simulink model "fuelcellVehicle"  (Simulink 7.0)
settings: Solver=ode45  StartTime=0.0  StopTime=10.0  RelTol=1e-3
InitFcn:
  | t_Start=tic;
StopFcn:
  | t_elapsed=toc(t_Start);
  | fuel_cons=(1000*(fueltank_simple1_std(end,1)/fueltank_simple1_std(end,3)))/(chassis_simple4_std(end,2)/100000);
  | 
  | disp(' ')
  | disp(['Time Elapsed: ' num2str(round(100*t_elapsed)/100) 's'])
  | disp(['Fuel Consumption: ' num2str(round(1000*fuel_cons)/1000) 'L/100km'])
undefined symbols (not defined in the file or in its folder): computed_mass, DC, fuelcellVehicle, Left, levelinit, slcm
libraries: simulink x11
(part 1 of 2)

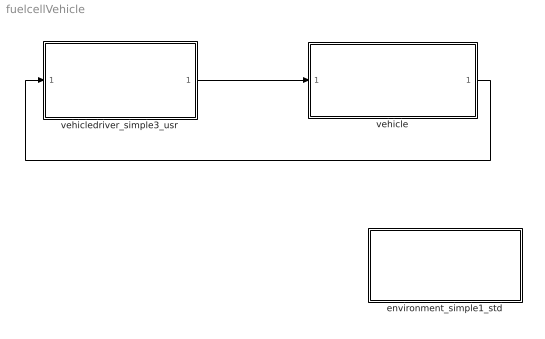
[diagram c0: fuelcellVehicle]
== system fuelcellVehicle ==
  environment_simple1_std : Subsystem  mask{Tamb=300, Pamb=101300}
      mask prompts: Tamb "Ambient Temperature [K]"; Pamb "Ambient Pressure [Pa]"
      mask help: Environment settings
  vehicle : Subsystem
  vehicledriver_simple3_usr : Subsystem  mask{Kp_driver=0.3, Ki_driver=0.02}
      mask prompts: Kp_driver "Proportional Gain"; Ki_driver "Integral Gain"
      mask help: Driver model
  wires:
  vehicledriver_simple3_usr/1(driver cmd out) -> vehicle/1(In1)
  vehicle/1(Out1) -> vehicledriver_simple3_usr/1(vehicle fb in)

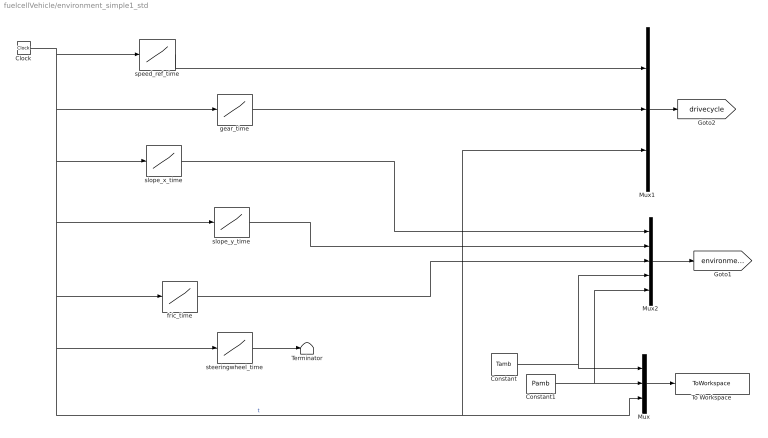
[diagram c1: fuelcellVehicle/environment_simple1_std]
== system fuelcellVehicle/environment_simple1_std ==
  Clock : Clock
  Constant : Constant  Value=Tamb  OutDataType=sfix(16)  OutScaling=2^0
  Constant1 : Constant  Value=Pamb  OutDataType=sfix(16)  OutScaling=2^0
  Mux : Mux  Inputs=3
  Mux1 : Mux  Inputs=3
  Mux2 : Mux  Inputs=5
  Terminator : Terminator
  To Workspace : ToWorkspace  VariableName=environment_simple1_std  SampleTime=-1  SaveFormat=Array
  fric_time : Lookup  InputValues=DC.time  Table=DC.fric  OutDataType=sfix(16)  OutScaling=2^0
  gear_time : Lookup  InputValues=DC.time  Table=DC.gearnr  OutDataType=sfix(16)  OutScaling=2^0
  slope_x_time : Lookup  InputValues=DC.time  Table=DC.slope_x  OutDataType=sfix(16)  OutScaling=2^0
  slope_y_time : Lookup  InputValues=DC.time  Table=DC.slope_y  OutDataType=sfix(16)  OutScaling=2^0
  speed_ref_time : Lookup  InputValues=DC.time  Table=DC.speed  OutDataType=sfix(16)  OutScaling=2^0
  steeringwheel_time : Lookup  InputValues=DC.time  Table=DC.steeringwheel  OutDataType=sfix(16)  OutScaling=2^0
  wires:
  Constant1/1 -> Mux/2, Mux2/5
  Constant/1 -> Mux/1, Mux2/4
  Mux/1 -> To Workspace/1
  Clock/1 -> speed_ref_time/1, gear_time/1, slope_x_time/1, slope_y_time/1, fric_time/1, Mux/3, Mux1/3, steeringwheel_time/1  "t"
  Mux1/1 -> [drivecycle]
  speed_ref_time/1 -> Mux1/1
  gear_time/1 -> Mux1/2
  slope_x_time/1 -> Mux2/1
  slope_y_time/1 -> Mux2/2
  fric_time/1 -> Mux2/3
  steeringwheel_time/1 -> Terminator/1
  Mux2/1 -> [environment]

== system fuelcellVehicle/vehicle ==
  In1 : Inport  OutDataType=sfix(16)  OutScaling=2^0
  Bus Creator : BusCreator  Orientation=up  Inputs=1
  Bus Creator1 : BusCreator  Orientation=up
  Bus Selector : BusSelector  Orientation=down  OutputSignals=fuelcell,electricmotor,chassis
  Ground : Ground
  Terminator : Terminator
  buffer_simple1_std : Subsystem
  chassis_simple4_std : Subsystem  InitFcn=computed_mass=calc_total_mass;
  controller_fuelcell1_usr : Subsystem  mask{SOCref=0.5}
      mask prompts: SOCref "SOC reference (0-1)"
      mask help: Main Controller
  electricmotor_quasistatic2_std : Subsystem
  electricsplit_simple1_std : Subsystem
  fuelcell_simple1_usr : Subsystem
  fueltank_simple1_std : Subsystem  mask{tanksize=??, level=100, fueldensity=??, Hf=??}
      mask prompts: tanksize "Size of fuel tank  [l]"; level "Level in tank [%]"; fueldensity "Fuel density [kg/m3]"; Hf "Specific Calorific Value [MJ/kg]"
      mask help: This is an ideal internal combustion engine component
  Out1 : Outport  OutDataType=sfix(16)  OutScaling=2^0
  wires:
  In1/1 -> controller_fuelcell1_usr/1(driver cmd in)
  controller_fuelcell1_usr/1(vehicle fb out) -> Out1/1
  electricmotor_quasistatic2_std/2(mech out [Nm]) -> chassis_simple4_std/2(mech in [Nm])
  chassis_simple4_std/2(mech fb out [rad/s]) -> electricmotor_quasistatic2_std/3(mech fb in [rad/s])
  fueltank_simple1_std/1(chem SCV out [MJ/kg]) -> fuelcell_simple1_usr/2(chem SCV in [MJ/kg])
  fuelcell_simple1_usr/3(chem fb out [kg/s]) -> fueltank_simple1_std/1(chem fb in [kg/s])
  controller_fuelcell1_usr/2(cmd out) -> Bus Selector/1
  Bus Creator1/1 -> controller_fuelcell1_usr/2(sensor in)
  Bus Creator/1 -> chassis_simple4_std/3(el in [V])
  chassis_simple4_std/3(el fb out [A]) -> Terminator/1
  Ground/1 -> Bus Creator/1  "voltage [V]"
  Bus Selector/1 -> fuelcell_simple1_usr/1(cmd)  "<fuelcell>"
  Bus Selector/2 -> electricmotor_quasistatic2_std/1(cmd in)  "<electricmotor>"
  Bus Selector/3 -> chassis_simple4_std/1(cmd)  "<chassis>"
  fuelcell_simple1_usr/1(sensor out) -> Bus Creator1/1
  electricmotor_quasistatic2_std/1(sensor out) -> Bus Creator1/2
  chassis_simple4_std/1(sensor out) -> Bus Creator1/3
  buffer_simple1_std/2(el out [V]) -> electricsplit_simple1_std/3(el split in [V])
  electricsplit_simple1_std/1(el out [V]) -> electricmotor_quasistatic2_std/2(el in [V])
  electricsplit_simple1_std/3(el split out [A]) -> buffer_simple1_std/1(el fb in [A])
  buffer_simple1_std/1(sensor out) -> Bus Creator1/4
  fuelcell_simple1_usr/2(el out [V]) -> electricsplit_simple1_std/1(el in [A])
  electricmotor_quasistatic2_std/3(el fb out [A]) -> electricsplit_simple1_std/2(el fb in [A])
  electricsplit_simple1_std/2(el fb out [V]) -> fuelcell_simple1_usr/3(el fb in [V])

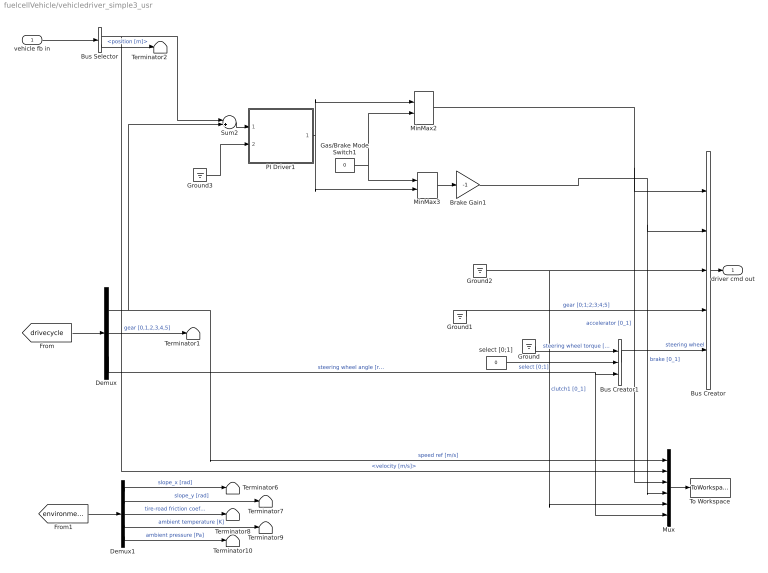
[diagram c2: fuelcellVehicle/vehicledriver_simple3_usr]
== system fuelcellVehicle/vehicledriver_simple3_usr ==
  vehicle fb in : Inport  OutDataType=sfix(16)  OutScaling=2^0
  Brake Gain1 : Gain  Gain=-1  ParameterDataType=sfix(16)  ParameterScaling=2^0  OutDataType=sfix(16)  OutScaling=2^0
  Bus Creator : BusCreator  Inputs=5
  Bus Creator1 : BusCreator  Inputs=3
  Bus Selector : BusSelector  OutputSignals=chassis.velocity [m/s],chassis.position [m]
  Demux : Demux  Outputs=3
  Demux1 : Demux  Outputs=5
  Gas/Brake Mode Switch1 : Constant  Value=0  OutDataType=sfix(16)  OutScaling=2^0
  Ground{,1..3} (4 alike) : Ground
  MinMax2 : MinMax  Function=max  Inputs=2  OutDataType=sfix(16)  OutScaling=2^0
  MinMax3 : MinMax  Inputs=2  OutDataType=sfix(16)  OutScaling=2^0
  Mux : Mux  Inputs=6
  PI Driver1 : Subsystem
  Sum2 : Sum  Inputs=-+  OutDataType=sfix(16)  OutScaling=2^0
  Terminator{1..2,6..10} (7 alike) : Terminator
  To Workspace : ToWorkspace  VariableName=driver_simple1_std  SampleTime=-1  SaveFormat=Array
  select [0;1] : Constant  Value=0  OutDataType=sfix(16)  OutScaling=2^0
  driver cmd out : Outport  OutDataType=sfix(16)  OutScaling=2^0
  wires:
  Ground3/1 -> PI Driver1/2(PI reset)
  select [0;1]/1 -> Bus Creator1/2  "select [0;1]"
  Demux/1 -> Sum2/2, Mux/1  "speed ref [m/s]"
  Demux/3 -> Bus Creator1/3, Mux/6  "steering wheel angle [rad]"
  [drivecycle] -> Demux/1
  Demux/2 -> Terminator1/1  "gear [0,1,2,3,4,5]"
  Demux1/5 -> Terminator10/1  "ambient pressure [Pa]"
  Demux1/4 -> Terminator9/1  "ambient temperature [K]"
  Demux1/1 -> Terminator6/1  "slope_x [rad]"
  Demux1/3 -> Terminator8/1  "tire-road friction coefficient [-]"
  [environment] -> Demux1/1
  Demux1/2 -> Terminator7/1  "slope_y [rad]"
  Bus Creator/1 -> driver cmd out/1
  Ground/1 -> Bus Creator1/1  "steering wheel torque [Nm]"
  Mux/1 -> To Workspace/1
  Bus Creator1/1 -> Bus Creator/5  "steering wheel"
  Ground1/1 -> Bus Creator/4  "gear [0;1;2;3;4;5]"
  Ground2/1 -> Bus Creator/3, Mux/5  "clutch1 [0_1]"
  MinMax2/1 -> Bus Creator/1, Mux/3  "accelerator [0_1]"
  Gas/Brake Mode Switch1/1 -> MinMax3/1, MinMax2/2
  MinMax3/1 -> Brake Gain1/1
  PI Driver1/1(PI out) -> MinMax3/2, MinMax2/1
  Brake Gain1/1 -> Bus Creator/2, Mux/4  "brake [0_1]"
  Sum2/1 -> PI Driver1/1(PI input)
  vehicle fb in/1 -> Bus Selector/1
  Bus Selector/1 -> Mux/2, Sum2/1  "<velocity [m/s]>"
  Bus Selector/2 -> Terminator2/1  "<position [m]>"

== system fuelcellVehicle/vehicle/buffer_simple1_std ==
  el fb in [A] : Inport  OutDataType=sfix(16)  OutScaling=2^0
  Model Info1 : Subsystem  LoadFcn=slcm LoadBlock;  InitFcn=slcm('UpdateAllCMBlocksInThisModelInit')  mask(CMBlock){InitialSaveTempField=, InitialBlockCM=None, BlockCM=None, Frame=on, SaveTempField=, DisplayStringWithTags=This model level is fixed. Place parameters in the subsystem masks, not on the top level., MaskDisplayString=This model level is fixed. Place parameters in the\nsubsystem masks, not on the top level., HorizontalTextAlignment=Left, LeftAlignmentValue=0.02, SourceBlockDiagram=fuelcellVehicle, TagMaxNumber=20, CMTag1=, CMTag2=, CMTag3=, CMTag4=, CMTag5=, CMTag6=, CMTag7=, CMTag8=, CMTag9=, CMTag10=, CMTag11=, CMTag12=, CMTag13=, CMTag14=, CMTag15=, CMTag16=, CMTag17=, CMTag18=, CMTag19=, CMTag20=}
      mask help: This block allows revision control information to be displayed within the model.
  buffer : Subsystem  mask{mass=??, Emax=??, Ri=??, Kvol=??, SOCinit=0.5}
      mask prompts: mass "Mass [kg]"; Emax "Maximum Energy level [J]"; Ri "Inner Resistance [Ohm]"; Kvol "Maximum voltage [V]"; SOCinit "SOC inital value"
      mask help: Electric buffer model
  local controller : Subsystem  mask{Kvol_c=??, Ri_c=??, Emax_c=??, SOCinit_c=??}
      mask prompts: Kvol_c "Maximum voltage [V]"; Ri_c "Inner Resistance [Ohm]"; Emax_c "Battery Energy Maxlevel [J]"; SOCinit_c "SOC initial level"
      mask help: Local controller for electric buffer
  sensor out : Outport  OutDataType=sfix(16)  OutScaling=2^0
  el out [V] : Outport  Port=2  OutDataType=sfix(16)  OutScaling=2^0
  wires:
  buffer/2(el out [V]) -> el out [V]/1
  local controller/1(sensor out) -> sensor out/1
  el fb in [A]/1 -> buffer/2(el fb in [A])
  buffer/1(sensor out) -> local controller/1(sensor in)
  local controller/2(ctrl) -> buffer/1(ctrl)

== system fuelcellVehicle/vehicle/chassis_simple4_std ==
  cmd : Inport  OutDataType=sfix(16)  OutScaling=2^0
  mech in [Nm] : Inport  Port=2  OutDataType=sfix(16)  OutScaling=2^0
  el in [V] : Inport  Port=3  OutDataType=sfix(16)  OutScaling=2^0
  chassis : Subsystem  mask{mass=??, nop=1, passengerweight=80, cargo=0, w_init=1, tirespec='205/55R16' %Modify this if needed, e=??, Cd=??, Af=??, rho=1.2, finalgear=3}
      mask prompts: mass "Chassis Mass [kg]"; nop "Number of passengers"; passengerweight "Weight of avg. passenger (kg)"; cargo "Cargo load (kg)"; w_init "Initial velocity [rad/s]"; tirespec "Tire specification (ex: '205/55R16')"; e "Rolling resistance coeff rear"; Cd "Air resistance cd (-)"; Af "Air resistance frontal area (m2)"; rho "Air density (kg/m3)"; finalgear "Final gear"
      mask help: Chassis model template
      mask init:
      | r=tireradius(tirespec);
  local controller : Subsystem
  sensor out : Outport  OutDataType=sfix(16)  OutScaling=2^0
  mech fb out [rad/s] : Outport  Port=2  OutDataType=sfix(16)  OutScaling=2^0
  el fb out [A] : Outport  Port=3  OutDataType=sfix(16)  OutScaling=2^0
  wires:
  local controller/2(ctrl) -> chassis/1(ctrl)
  chassis/2(mech fb out [rad/s]) -> mech fb out [rad/s]/1
  mech in [Nm]/1 -> chassis/2(mech in [Nm])
  chassis/1(sensor out) -> local controller/2(sensor in)
  local controller/1(sensor out) -> sensor out/1
  cmd/1 -> local controller/1(cmd in)
  el in [V]/1 -> chassis/3(el in [V])
  chassis/3(el fb out [A]) -> el fb out [A]/1

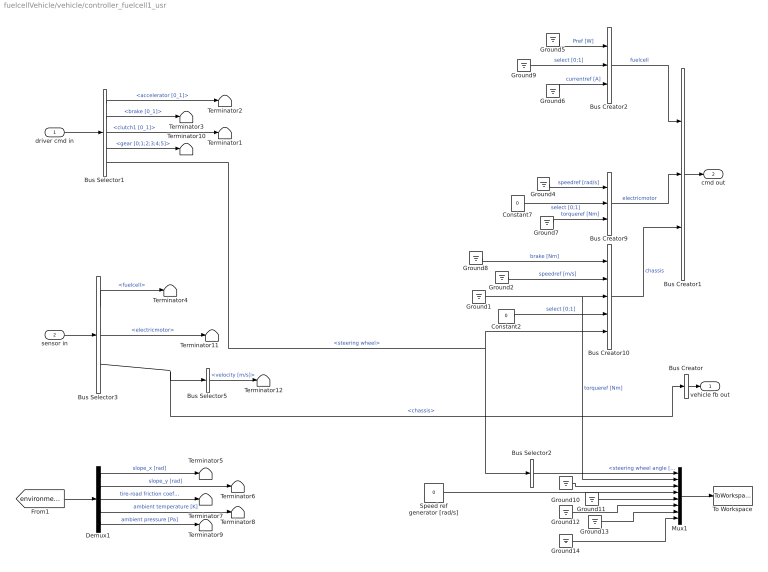
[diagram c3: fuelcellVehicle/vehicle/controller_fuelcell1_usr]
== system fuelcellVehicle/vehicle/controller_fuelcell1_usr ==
  driver cmd in : Inport  OutDataType=sfix(16)  OutScaling=2^0
  sensor in : Inport  Port=2  OutDataType=sfix(16)  OutScaling=2^0
  Bus Creator : BusCreator  Inputs=1
  Bus Creator1 : BusCreator  Inputs=3
  Bus Creator10 : BusCreator  Inputs=5
  Bus Creator2 : BusCreator  Inputs=3
  Bus Creator9 : BusCreator  Inputs=3
  Bus Selector1 : BusSelector  OutputSignals=accelerator [0_1],brake [0_1],clutch1 [0_1],gear [0;1;2;3;4;5],steering wheel
  Bus Selector2 : BusSelector  OutputSignals=steering wheel angle [rad]
  Bus Selector3 : BusSelector  OutputSignals=fuelcell,electricmotor,chassis
  Bus Selector5 : BusSelector  OutputSignals=velocity [m/s]
  Constant2 : Constant  Value=0  OutDataType=sfix(16)  OutScaling=2^0
  Constant7 : Constant  Value=0  OutDataType=sfix(16)  OutScaling=2^0
  Demux1 : Demux  Outputs=5
  Ground{1..2,4..14} (13 alike) : Ground
  Mux1 : Mux  Inputs=8
  Speed ref generator [rad/s] : Constant  Value=0  OutDataType=sfix(16)  OutScaling=2^0
  Terminator{1..12} (12 alike) : Terminator
  To Workspace : ToWorkspace  VariableName=controller_fuelcell1_usr  SampleTime=-1  SaveFormat=Array
  vehicle fb out : Outport  OutDataType=sfix(16)  OutScaling=2^0
  cmd out : Outport  Port=2  OutDataType=sfix(16)  OutScaling=2^0
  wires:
  Demux1/5 -> Terminator9/1  "ambient pressure [Pa]"
  Demux1/4 -> Terminator8/1  "ambient temperature [K]"
  Demux1/1 -> Terminator5/1  "slope_x [rad]"
  Demux1/3 -> Terminator7/1  "tire-road friction coefficient [-]"
  [environment] -> Demux1/1
  Demux1/2 -> Terminator6/1  "slope_y [rad]"
  Speed ref generator [rad/s]/1 -> Mux1/4
  Bus Selector2/1 -> Mux1/1  "<steering wheel angle [rad]>"
  Mux1/1 -> To Workspace/1
  Constant2/1 -> Bus Creator10/4  "select [0;1]"
  Ground1/1 -> Mux1/2, Bus Creator10/3  "torqueref [Nm]"
  Ground2/1 -> Bus Creator10/2  "speedref [m/s]"
  Bus Creator10/1 -> Bus Creator1/3  "chassis"
  Bus Creator9/1 -> Bus Creator1/2  "electricmotor"
  Constant7/1 -> Bus Creator9/2  "select [0;1]"
  Ground4/1 -> Bus Creator9/1  "speedref [rad/s]"
  Bus Selector3/3 -> Bus Creator/1, Bus Selector5/1  "<chassis>"
  Bus Selector3/1 -> Terminator4/1  "<fuelcell>"
  Bus Selector3/2 -> Terminator11/1  "<electricmotor>"
  sensor in/1 -> Bus Selector3/1
  driver cmd in/1 -> Bus Selector1/1
  Bus Selector1/5 -> Bus Selector2/1, Bus Creator10/5  "<steering wheel>"
  Bus Creator/1 -> vehicle fb out/1
  Bus Creator1/1 -> cmd out/1
  Bus Creator2/1 -> Bus Creator1/1  "fuelcell"
  Ground5/1 -> Bus Creator2/1  "Pref [W]"
  Ground6/1 -> Bus Creator2/3  "currentref [A]"
  Bus Selector1/2 -> Terminator3/1  "<brake [0_1]>"
  Bus Selector1/1 -> Terminator2/1  "<accelerator [0_1]>"
  Bus Selector1/3 -> Terminator1/1  "<clutch1 [0_1]>"
  Bus Selector1/4 -> Terminator10/1  "<gear [0;1;2;3;4;5]>"
  Ground7/1 -> Bus Creator9/3  "torqueref [Nm]"
  Ground8/1 -> Bus Creator10/1  "brake [Nm]"
  Ground9/1 -> Bus Creator2/2  "select [0;1]"
  Bus Selector5/1 -> Terminator12/1  "<velocity [m/s]>"
  Ground10/1 -> Mux1/3
  Ground11/1 -> Mux1/5
  Ground12/1 -> Mux1/6
  Ground13/1 -> Mux1/7
  Ground14/1 -> Mux1/8

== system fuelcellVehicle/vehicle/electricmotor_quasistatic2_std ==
  cmd in : Inport  OutDataType=sfix(16)  OutScaling=2^0
  el in [V] : Inport  Port=2  OutDataType=sfix(16)  OutScaling=2^0
  mech fb in [rad/s] : Inport  Port=3  OutDataType=sfix(16)  OutScaling=2^0
  electricmotor : Subsystem  mask{mass=??, inertia=??, ka=??, ki=??, R=??}
      mask prompts: mass "Mass (kg)"; inertia "Inertia (kg*m^2)"; ka "Motor torque constant (Nm/A) (slightly smaller than voltage/speed constant)"; ki "Voltage/speed constant"; R "Resistance (ohm)"
  local controller : Subsystem  mask{kac=??, kic=??, Rc=??, Pmax=??, Kp=10, Ki=1}
      mask prompts: kac "Motor torque constant (Nm/A) (slightly smaller than voltage/speed constant)"; kic "Voltage/speed constant"; Rc "Motor resistance (ohm)"; Pmax "Max power (kW)"; Kp "Speed controller (Kp)"; Ki "Speed controller (Ki)"
  sensor out : Outport  OutDataType=sfix(16)  OutScaling=2^0
  mech out [Nm] : Outport  Port=2  OutDataType=sfix(16)  OutScaling=2^0
  el fb out [A] : Outport  Port=3  OutDataType=sfix(16)  OutScaling=2^0
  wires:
  local controller/1(sensor out) -> sensor out/1
  electricmotor/2(mech power out [Nm]) -> mech out [Nm]/1
  electricmotor/3(el fb out [A]) -> el fb out [A]/1
  cmd in/1 -> local controller/1(cmd in)
  mech fb in [rad/s]/1 -> electricmotor/3(mech fb in [rad/s])
  el in [V]/1 -> electricmotor/2(el power in [V])
  electricmotor/1(sensor out) -> local controller/2(sensor in)
  local controller/2(ctrl out) -> electricmotor/1(ctrl in)

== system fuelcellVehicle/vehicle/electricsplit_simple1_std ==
  el in [A] : Inport  OutDataType=sfix(16)  OutScaling=2^0
  el fb in [A] : Inport  Port=2  OutDataType=sfix(16)  OutScaling=2^0
  el split in [V] : Inport  Port=3  OutDataType=sfix(16)  OutScaling=2^0
  Model Info1 : simulink/Model-Wide Utilities/Model Info  SystemSampleTime=-1  InitialBlockCM=None  BlockCM=None  Frame=on  DisplayStringWithTags=This model level is fixed. Place parameters in the subsystem masks, not on the top level.  HorizontalTextAlignment=Left  LeftAlignmentValue=0.02  SourceBlockDiagram=fuelcellVehicle  TagMaxNumber=20
  electricsplit : Subsystem  mask{mass=0}
      mask prompts: mass "Mass [kg]"
      mask help: Electric buffer template model
  local controller : Subsystem
  el out [V] : Outport  OutDataType=sfix(16)  OutScaling=2^0
  el fb out [V] : Outport  Port=2  OutDataType=sfix(16)  OutScaling=2^0
  el split out [A] : Outport  Port=3  OutDataType=sfix(16)  OutScaling=2^0
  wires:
  local controller/1(ctrl) -> electricsplit/1(ctrl)
  electricsplit/1(sensor out) -> local controller/1(sensor in)
  el split in [V]/1 -> electricsplit/4(el split in [V])
  electricsplit/4(el split out [A]) -> el split out [A]/1
  el in [A]/1 -> electricsplit/2(el in [A])
  el fb in [A]/1 -> electricsplit/3(el fb in [A])
  electricsplit/3(el fb out [V]) -> el fb out [V]/1
  electricsplit/2(el out [V]) -> el out [V]/1

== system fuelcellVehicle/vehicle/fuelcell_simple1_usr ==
  cmd : Inport  OutDataType=sfix(16)  OutScaling=2^0
  chem SCV in [MJ/kg] : Inport  Port=2  OutDataType=sfix(16)  OutScaling=2^0
  el fb in [V] : Inport  Port=3  OutDataType=sfix(16)  OutScaling=2^0
  Model Info1 : Subsystem  LoadFcn=slcm LoadBlock;  InitFcn=slcm('UpdateAllCMBlocksInThisModelInit')  mask(CMBlock){InitialSaveTempField=, InitialBlockCM=None, BlockCM=None, Frame=on, SaveTempField=, DisplayStringWithTags=This model level is fixed. Place parameters in the subsystem masks, not on the top level., MaskDisplayString=This model level is fixed. Place parameters in the\nsubsystem masks, not on the top level., HorizontalTextAlignment=Left, LeftAlignmentValue=0.02, SourceBlockDiagram=fuelcellVehicle, TagMaxNumber=20, CMTag1=, CMTag2=, CMTag3=, CMTag4=, CMTag5=, CMTag6=, CMTag7=, CMTag8=, CMTag9=, CMTag10=, CMTag11=, CMTag12=, CMTag13=, CMTag14=, CMTag15=, CMTag16=, CMTag17=, CMTag18=, CMTag19=, CMTag20=}
      mask help: This block allows revision control information to be displayed within the model.
  fuelcell : Subsystem  mask{mass=??}
      mask prompts: mass "Mass [kg]"
      mask help: Internal combustion engine template model
  local controller : Subsystem
  sensor out : Outport  OutDataType=sfix(16)  OutScaling=2^0
  el out [V] : Outport  Port=2  OutDataType=sfix(16)  OutScaling=2^0
  chem fb out [kg/s] : Outport  Port=3  OutDataType=sfix(16)  OutScaling=2^0
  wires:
  fuelcell/2(el power out [A]) -> el out [V]/1
  el fb in [V]/1 -> fuelcell/3(el fb in [V])
  fuelcell/1(sensor out) -> local controller/2(sensor in)
  local controller/1(sensor out) -> sensor out/1
  cmd/1 -> local controller/1(cmd)
  local controller/2(ctrl) -> fuelcell/1(ctrl)
  fuelcell/3(chem fb out [kg/s]) -> chem fb out [kg/s]/1
  chem SCV in [MJ/kg]/1 -> fuelcell/2(chem SCV in [MJ/kg])

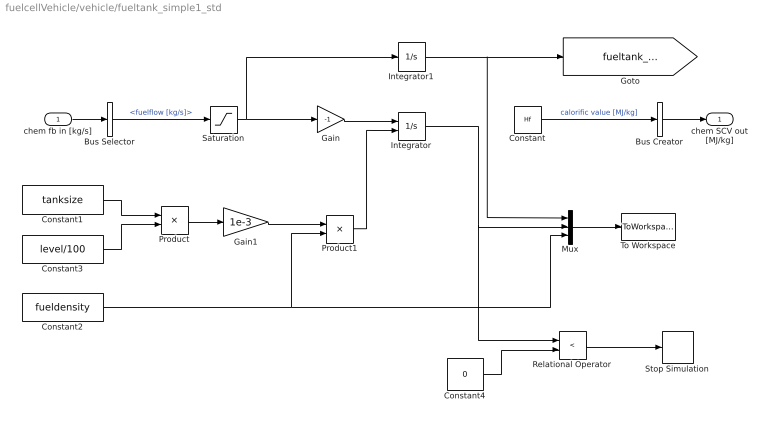
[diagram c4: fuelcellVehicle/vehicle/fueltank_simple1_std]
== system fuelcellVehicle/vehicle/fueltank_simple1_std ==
  chem fb in [kg/s] : Inport  OutDataType=sfix(16)  OutScaling=2^0
  Bus Creator : BusCreator  Inputs=1
  Bus Selector : BusSelector  OutputSignals=fuelflow [kg/s]
  Constant : Constant  Value=Hf  OutDataType=sfix(16)  OutScaling=2^0
  Constant1 : Constant  Value=tanksize  OutDataType=sfix(16)  OutScaling=2^0
  Constant2 : Constant  Value=fueldensity  OutDataType=sfix(16)  OutScaling=2^0
  Constant3 : Constant  Value=level/100  OutDataType=sfix(16)  OutScaling=2^0
  Constant4 : Constant  Value=0  OutDataType=sfix(16)  OutScaling=2^0
  Gain : Gain  Gain=-1  ParameterDataType=sfix(16)  ParameterScaling=2^0  OutDataType=sfix(16)  OutScaling=2^0
  Gain1 : Gain  Gain=1e-3  ParameterDataType=sfix(16)  ParameterScaling=2^0  OutDataType=sfix(16)  OutScaling=2^0
  Integrator : Integrator  InitialConditionSource=external  InitialCondition=levelinit
  Integrator1 : Integrator
  Mux : Mux  Inputs=3
  Product : Product  OutDataType=sfix(16)  OutScaling=2^0
  Product1 : Product  OutDataType=sfix(16)  OutScaling=2^0
  Relational Operator : RelationalOperator  Operator=<  LogicOutDataTypeMode=boolean
  Saturation : Saturate  UpperLimit=inf  LowerLimit=0
  Stop Simulation : Stop
  To Workspace : ToWorkspace  VariableName=fueltank_simple1_std  SampleTime=-1  SaveFormat=Array
  chem SCV out [MJ/kg] : Outport  OutDataType=sfix(16)  OutScaling=2^0
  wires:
  chem fb in [kg/s]/1 -> Bus Selector/1
  Constant/1 -> Bus Creator/1  "calorific value [MJ/kg]"
  Gain/1 -> Integrator/1
  Bus Selector/1 -> Saturation/1  "<fuelflow [kg/s]>"
  Mux/1 -> To Workspace/1
  Integrator1/1 -> Mux/1, [fueltank_weight_reduction]
  Integrator/1 -> Mux/2, Relational Operator/1
  Bus Creator/1 -> chem SCV out [MJ/kg]/1
  Constant1/1 -> Product/1
  Constant3/1 -> Product/2
  Constant2/1 -> Mux/3, Product1/2
  Product/1 -> Gain1/1
  Product1/1 -> Integrator/2
  Gain1/1 -> Product1/1
  Constant4/1 -> Relational Operator/2
  Relational Operator/1 -> Stop Simulation/1
  Saturation/1 -> Gain/1, Integrator1/1

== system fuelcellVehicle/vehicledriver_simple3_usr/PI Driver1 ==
  PI input : Inport  OutDataType=sfix(16)  OutScaling=2^0
  PI reset : Inport  Port=2  OutDataType=sfix(16)  OutScaling=2^0
  Integrator : Integrator  ExternalReset=either  LimitOutput=on  UpperSaturationLimit=30  LowerSaturationLimit=0
  Ki : Gain  Gain=Ki_driver  ParameterDataType=sfix(16)  ParameterScaling=2^0  OutDataType=sfix(16)  OutScaling=2^0
  Kp : Gain  Gain=Kp_driver  ParameterDataType=sfix(16)  ParameterScaling=2^0  OutDataType=sfix(16)  OutScaling=2^0
  Saturation : Saturate  UpperLimit=1  LowerLimit=-1
  Sum : Sum  Inputs=|++  OutDataType=sfix(16)  OutScaling=2^0
  PI out : Outport  OutDataType=sfix(16)  OutScaling=2^0
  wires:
  Kp/1 -> Sum/1
  PI reset/1 -> Integrator/2
  Saturation/1 -> PI out/1
  Sum/1 -> Saturation/1
  Ki/1 -> Sum/2
  Integrator/1 -> Ki/1
  PI input/1 -> Kp/1, Integrator/1

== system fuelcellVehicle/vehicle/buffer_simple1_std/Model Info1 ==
  EmptySubsystem : Subsystem

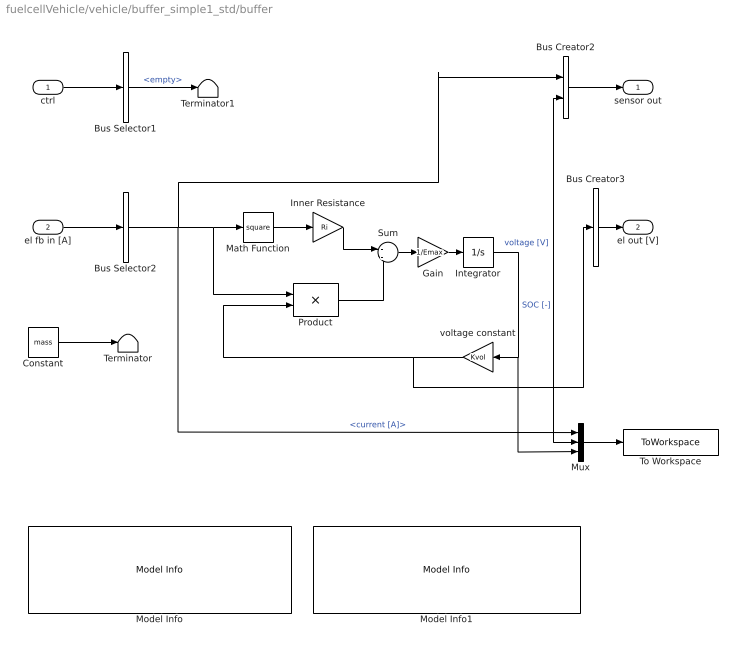
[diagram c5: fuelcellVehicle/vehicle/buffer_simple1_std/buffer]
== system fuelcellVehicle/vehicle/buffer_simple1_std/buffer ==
  ctrl : Inport  OutDataType=sfix(16)  OutScaling=2^0
  el fb in [A] : Inport  Port=2  OutDataType=sfix(16)  OutScaling=2^0
  Bus Creator2 : BusCreator  Inputs=2
  Bus Creator3 : BusCreator  Inputs=1
  Bus Selector1 : BusSelector  OutputSignals=empty
  Bus Selector2 : BusSelector  OutputSignals=current [A]
  Constant : Constant  Value=mass  OutDataType=sfix(16)  OutScaling=2^0
  Gain : Gain  Gain=1/Emax  ParameterDataType=sfix(16)  ParameterScaling=2^0  OutDataType=sfix(16)  OutScaling=2^0
  Inner Resistance : Gain  Gain=Ri  ParameterDataType=sfix(16)  ParameterScaling=2^0  OutDataType=sfix(16)  OutScaling=2^0
  Integrator : Integrator  InitialCondition=SOCinit  LimitOutput=on  UpperSaturationLimit=1  LowerSaturationLimit=0
  Math Function : Math  Operator=square  OutDataType=sfix(16)  OutScaling=2^0
  Model Info : simulink/Model-Wide Utilities/Model Info  SystemSampleTime=-1  InitialBlockCM=None  BlockCM=None  Frame=on  DisplayStringWithTags=|  HorizontalTextAlignment=Left  LeftAlignmentValue=0.02  SourceBlockDiagram=fuelcellVehicle  TagMaxNumber=20
      | Modified: %<ModifiedDate>
      | 
      | The nodes "ctrl" and "sensor out" must conform 
      | with the corresponding nodes of the local controller. 
      | The other nodes are fixed.
  Model Info1 : simulink/Model-Wide Utilities/Model Info  SystemSampleTime=-1  InitialBlockCM=None  BlockCM=None  Frame=on  DisplayStringWithTags=Your own comments!  HorizontalTextAlignment=Left  LeftAlignmentValue=0.02  SourceBlockDiagram=fuelcellVehicle  TagMaxNumber=20
  Mux : Mux  Inputs=3
  Product : Product  OutDataType=sfix(16)  OutScaling=2^0
  Sum : Sum  Inputs=-|-  OutDataType=sfix(16)  OutScaling=2^0
  Terminator : Terminator
  Terminator1 : Terminator
  To Workspace : ToWorkspace  VariableName=buffer_simple1_std  SampleTime=-1  SaveFormat=Array
  voltage constant : Gain  Orientation=left  Gain=Kvol  ParameterDataType=sfix(16)  ParameterScaling=2^0  OutDataType=sfix(16)  OutScaling=2^0
  sensor out : Outport  OutDataType=sfix(16)  OutScaling=2^0
  el out [V] : Outport  Port=2  OutDataType=sfix(16)  OutScaling=2^0
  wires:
  Bus Selector1/1 -> Terminator1/1  "<empty>"
  ctrl/1 -> Bus Selector1/1
  Bus Creator2/1 -> sensor out/1
  Bus Creator3/1 -> el out [V]/1
  Bus Selector2/1 -> Bus Creator2/1, Math Function/1, Product/1, Mux/1  "<current [A]>"
  el fb in [A]/1 -> Bus Selector2/1
  Constant/1 -> Terminator/1
  Integrator/1 -> voltage constant/1, Mux/3  "SOC [-]"
  Gain/1 -> Integrator/1
  Math Function/1 -> Inner Resistance/1
  voltage constant/1 -> Product/2, Bus Creator3/1, Bus Creator2/2, Mux/2  "voltage [V]"
  Inner Resistance/1 -> Sum/1
  Product/1 -> Sum/2
  Sum/1 -> Gain/1
  Mux/1 -> To Workspace/1

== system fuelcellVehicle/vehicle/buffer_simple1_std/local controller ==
  sensor in : Inport  OutDataType=sfix(16)  OutScaling=2^0
  Bus Creator1 : BusCreator  Inputs=1
  Bus Creator2 : BusCreator  Inputs=3
  Bus Selector2 : BusSelector  OutputSignals=current [A],voltage [V]
  Ground : Ground
  Model Info : simulink/Model-Wide Utilities/Model Info  SystemSampleTime=-1  InitialBlockCM=None  BlockCM=None  Frame=on  DisplayStringWithTags=|  HorizontalTextAlignment=Left  LeftAlignmentValue=0.02  SourceBlockDiagram=fuelcellVehicle  TagMaxNumber=20
      | Modified: %<ModifiedDate>
      | 
      | The nodes "cmd in" and "sensor out" are fixed.
      | The nodes "sensor in" and "ctrl", however, 
      | may be adjusted arbitrarily since the local controller is 
      | made specifically for a certain component model.
  Model Info1 : simulink/Model-Wide Utilities/Model Info  SystemSampleTime=-1  InitialBlockCM=None  BlockCM=None  Frame=on  DisplayStringWithTags=Your own comments!  HorizontalTextAlignment=Left  LeftAlignmentValue=0.02  SourceBlockDiagram=fuelcellVehicle  TagMaxNumber=20
  SOC estimator : Subsystem
  sensor out : Outport  OutDataType=sfix(16)  OutScaling=2^0
  ctrl : Outport  Port=2  OutDataType=sfix(16)  OutScaling=2^0
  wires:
  Bus Selector2/2 -> Bus Creator2/3  "<voltage [V]>"
  Ground/1 -> Bus Creator1/1  "empty"
  Bus Creator1/1 -> ctrl/1
  Bus Creator2/1 -> sensor out/1  "buffer"
  Bus Selector2/1 -> Bus Creator2/1, SOC estimator/1(current in)  "<current [A]>"
  sensor in/1 -> Bus Selector2/1
  SOC estimator/1(SOC) -> Bus Creator2/2  "SOC [-]"

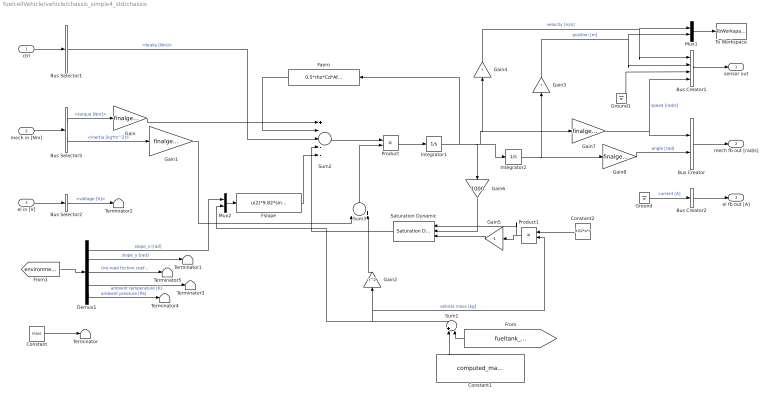
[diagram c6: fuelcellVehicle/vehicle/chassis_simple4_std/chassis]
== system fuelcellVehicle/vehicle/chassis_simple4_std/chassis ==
  ctrl : Inport  OutDataType=sfix(16)  OutScaling=2^0
  mech in [Nm] : Inport  Port=2  OutDataType=sfix(16)  OutScaling=2^0
  el in [V] : Inport  Port=3  OutDataType=sfix(16)  OutScaling=2^0
  Bus Creator : BusCreator  Inputs=2
  Bus Creator1 : BusCreator
  Bus Creator2 : BusCreator  Inputs=1
  Bus Selector1 : BusSelector  OutputSignals=brake [Nm]
  Bus Selector2 : BusSelector  OutputSignals=voltage [V]
  Bus Selector5 : BusSelector  OutputSignals=torque [Nm],inertia [kg*m^2]
  Constant : Constant  Value=mass  OutDataType=sfix(16)  OutScaling=2^0
  Constant1 : Constant  Orientation=up  Value=computed_mass  OutDataType=sfix(16)  OutScaling=2^0
  Constant2 : Constant  Orientation=left  Value=9.82*e*r  OutDataType=sfix(16)  OutScaling=2^0
  Demux1 : Demux  Outputs=5
  Faero : Fcn  Orientation=left  Expr=0.5*rho*Cd*Af*u^2*r^3
  Fslope : Fcn  Expr=u(2)*9.82*sin(u(1))
  Gain : Gain  Gain=finalgear  ParameterDataType=sfix(16)  ParameterScaling=2^0  OutDataType=sfix(16)  OutScaling=2^0
  Gain1 : Gain  Gain=finalgear^2  ParameterDataType=sfix(16)  ParameterScaling=2^0  OutDataType=sfix(16)  OutScaling=2^0
  Gain2 : Gain  Orientation=up  Gain=r^2  ParameterDataType=sfix(16)  ParameterScaling=2^0  OutDataType=sfix(16)  OutScaling=2^0
  Gain3 : Gain  Orientation=up  Gain=r  ParameterDataType=sfix(16)  ParameterScaling=2^0  OutDataType=sfix(16)  OutScaling=2^0
  Gain4 : Gain  Orientation=up  Gain=r  ParameterDataType=sfix(16)  ParameterScaling=2^0  OutDataType=sfix(16)  OutScaling=2^0
  Gain5 : Gain  Orientation=left  Gain=-1  ParameterDataType=sfix(16)  ParameterScaling=2^0  OutDataType=sfix(16)  OutScaling=2^0
  Gain6 : Gain  Orientation=down  Gain=1000  ParameterDataType=sfix(16)  ParameterScaling=2^0  OutDataType=sfix(16)  OutScaling=2^0
  Gain7 : Gain  Gain=finalgear  ParameterDataType=sfix(16)  ParameterScaling=2^0  OutDataType=sfix(16)  OutScaling=2^0
  Gain8 : Gain  Gain=finalgear  ParameterDataType=sfix(16)  ParameterScaling=2^0  OutDataType=sfix(16)  OutScaling=2^0
  Ground : Ground
  Ground1 : Ground
  Integrator1 : Integrator  InitialCondition=w_init
  Integrator2 : Integrator
  Mux1 : Mux  Inputs=2
  Mux2 : Mux  Inputs=2
  Product : Product  Inputs=*/  OutDataType=sfix(16)  OutScaling=2^0
  Product1 : Product  Orientation=left  Inputs=**  OutDataType=sfix(16)  OutScaling=2^0
  Saturation Dynamic : simulink/Discontinuities/Saturation Dynamic  Orientation=left  SystemSampleTime=-1  OutMin=[]  OutMax=[]  OutDataTypeStr=Inherit: Same as second input  OutDataType=sfix(16)  OutScaling=2^-10  DoSatur=off
  Sum1 : Sum  Orientation=up  Inputs=+|-  OutDataType=sfix(16)  OutScaling=2^0
  Sum2 : Sum  Inputs=+----  OutDataType=sfix(16)  OutScaling=2^0
  Sum3 : Sum  Orientation=up  OutDataType=sfix(16)  OutScaling=2^0
  Terminator{,1..5} (6 alike) : Terminator
  To Workspace : ToWorkspace  VariableName=chassis_simple4_std  SampleTime=-1  SaveFormat=Array
  sensor out : Outport  OutDataType=sfix(16)  OutScaling=2^0
  mech fb out [rad/s] : Outport  Port=2  OutDataType=sfix(16)  OutScaling=2^0
  el fb out [A] : Outport  Port=3  OutDataType=sfix(16)  OutScaling=2^0
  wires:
  Ground1/1 -> Bus Creator1/3
  Mux2/1 -> Fslope/1
  Bus Selector5/2 -> Gain1/1  "<inertia [kg*m^2]>"
  Bus Selector5/1 -> Gain/1  "<torque [Nm]>"
  Bus Creator/1 -> mech fb out [rad/s]/1
  mech in [Nm]/1 -> Bus Selector5/1
  Constant/1 -> Terminator/1
  Bus Creator1/1 -> sensor out/1
  Mux1/1 -> To Workspace/1
  ctrl/1 -> Bus Selector1/1
  Bus Selector2/1 -> Terminator2/1  "<voltage [V]>"
  el in [V]/1 -> Bus Selector2/1
  Bus Creator2/1 -> el fb out [A]/1
  Ground/1 -> Bus Creator2/1  "current [A]"
  Constant1/1 -> Sum1/1
  Sum1/1 -> Mux2/2, Gain2/1, Product1/2  "vehicle mass [kg]"
  [fueltank_weight_reduction] -> Sum1/2
  Demux1/2 -> Terminator1/1  "slope_y [rad]"
  [environment] -> Demux1/1
  Demux1/4 -> Terminator3/1  "ambient temperature [K]"
  Demux1/5 -> Terminator4/1  "ambient pressure [Pa]"
  Demux1/3 -> Terminator5/1  "tire-road friction coefficient [-]"
  Bus Selector1/1 -> Sum2/3  "<brake [Nm]>"
  Demux1/1 -> Mux2/1  "slope_x [rad]"
  Gain/1 -> Sum2/1
  Integrator1/1 -> Faero/1, Integrator2/1, Gain4/1, Gain7/1, Gain6/1
  Faero/1 -> Sum2/2
  Fslope/1 -> Sum2/5
  Integrator2/1 -> Gain3/1, Gain8/1
  Gain2/1 -> Sum3/2
  Gain1/1 -> Sum3/1
  Sum3/1 -> Product/2
  Product/1 -> Integrator1/1
  Sum2/1 -> Product/1
  Gain3/1 -> Mux1/2, Bus Creator1/2  "position [m]"
  Gain4/1 -> Mux1/1, Bus Creator1/1  "velocity [m/s]"
  Saturation Dynamic/1 -> Sum2/4
  Product1/1 -> Gain5/1, Saturation Dynamic/1
  Constant2/1 -> Product1/1
  Gain5/1 -> Saturation Dynamic/3
  Gain6/1 -> Saturation Dynamic/2
  Gain7/1 -> Bus Creator/1, Bus Creator1/4  "speed [rad/s]"
  Gain8/1 -> Bus Creator/2  "angle [rad]"

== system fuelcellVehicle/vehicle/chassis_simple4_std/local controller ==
  cmd in : Inport  OutDataType=sfix(16)  OutScaling=2^0
  sensor in : Inport  Port=2  OutDataType=sfix(16)  OutScaling=2^0
  Bus Creator1 : BusCreator  Inputs=1
  Bus Creator2 : BusCreator  Inputs=2
  Bus Selector1 : BusSelector  OutputSignals=velocity [m/s],position [m]
  Bus Selector2 : BusSelector  OutputSignals=brake [Nm]
  sensor out : Outport  OutDataType=sfix(16)  OutScaling=2^0
  ctrl : Outport  Port=2  OutDataType=sfix(16)  OutScaling=2^0
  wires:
  Bus Selector2/1 -> Bus Creator1/1  "<brake [Nm]>"
  Bus Creator1/1 -> ctrl/1
  Bus Creator2/1 -> sensor out/1  "chassis"
  sensor in/1 -> Bus Selector1/1
  Bus Selector1/1 -> Bus Creator2/1  "<velocity [m/s]>"
  cmd in/1 -> Bus Selector2/1
  Bus Selector1/2 -> Bus Creator2/2  "<position [m]>"

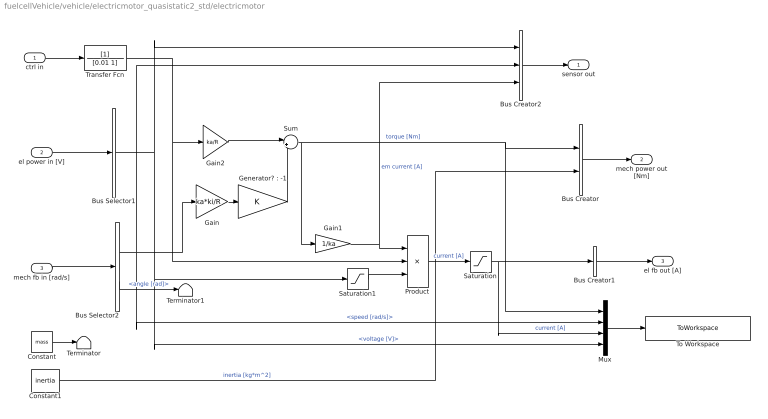
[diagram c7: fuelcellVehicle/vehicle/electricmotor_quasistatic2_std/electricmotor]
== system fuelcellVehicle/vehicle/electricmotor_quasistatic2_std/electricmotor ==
  ctrl in : Inport  OutDataType=sfix(16)  OutScaling=2^0
  el power in [V] : Inport  Port=2  OutDataType=sfix(16)  OutScaling=2^0
  mech fb in [rad/s] : Inport  Port=3  OutDataType=sfix(16)  OutScaling=2^0
  Bus Creator : BusCreator  Inputs=2
  Bus Creator1 : BusCreator  Inputs=1
  Bus Creator2 : BusCreator  Inputs=3
  Bus Selector1 : BusSelector  OutputSignals=voltage [V]
  Bus Selector2 : BusSelector  OutputSignals=speed [rad/s],angle [rad]
  Constant : Constant  Value=mass  OutDataType=sfix(16)  OutScaling=2^0
  Constant1 : Constant  Value=inertia  OutDataType=sfix(16)  OutScaling=2^0
  Gain : Gain  Gain=ka*ki/R  ParameterDataType=sfix(16)  ParameterScaling=2^0  OutDataType=sfix(16)  OutScaling=2^0
  Gain1 : Gain  Gain=1/ka  ParameterDataType=sfix(16)  ParameterScaling=2^0  OutDataType=sfix(16)  OutScaling=2^0
  Gain2 : Gain  Gain=ka/R  ParameterDataType=sfix(16)  ParameterScaling=2^0  OutDataType=sfix(16)  OutScaling=2^0
  "Generator? : -1" : Gain  ParameterDataType=sfix(16)  ParameterScaling=2^0  OutDataType=sfix(16)  OutScaling=2^0
  Mux : Mux
  Product : Product  Inputs=**/  OutDataType=sfix(16)  OutScaling=2^0
  Saturation : Saturate  UpperLimit=300  LowerLimit=-300
  Saturation1 : Saturate  UpperLimit=inf  LowerLimit=0.1
  Sum : Sum  Inputs=|+-  OutDataType=sfix(16)  OutScaling=2^0
  Terminator : Terminator
  Terminator1 : Terminator
  To Workspace : ToWorkspace  VariableName=electricmotor_quasistatic2_std  SampleTime=-1  SaveFormat=Array
  Transfer Fcn : TransferFcn  Denominator=[0.01 1]
  sensor out : Outport  OutDataType=sfix(16)  OutScaling=2^0
  mech power out [Nm] : Outport  Port=2  OutDataType=sfix(16)  OutScaling=2^0
  el fb out [A] : Outport  Port=3  OutDataType=sfix(16)  OutScaling=2^0
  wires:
  Bus Creator1/1 -> el fb out [A]/1
  Bus Selector2/2 -> Terminator1/1  "<angle [rad]>"
  Bus Creator/1 -> mech power out [Nm]/1
  el power in [V]/1 -> Bus Selector1/1
  Constant/1 -> Terminator/1
  mech fb in [rad/s]/1 -> Bus Selector2/1
  ctrl in/1 -> Transfer Fcn/1
  Bus Selector2/1 -> Mux/2, Gain/1, Bus Creator2/2  "<speed [rad/s]>"
  Bus Selector1/1 -> Bus Creator2/1, Mux/4, Saturation1/1  "<voltage [V]>"
  Product/1 -> Saturation/1  "current [A]"
  Mux/1 -> To Workspace/1
  Bus Creator2/1 -> sensor out/1
  Constant1/1 -> Bus Creator/2  "inertia [kg*m^2]"
  Gain/1 -> "Generator? : -1"/1
  Gain1/1 -> Bus Creator2/3, Product/1  "em current [A]"
  Transfer Fcn/1 -> Gain2/1, Product/2
  Gain2/1 -> Sum/1
  Sum/1 -> Gain1/1, Mux/1, Bus Creator/1  "torque [Nm]"
  "Generator? : -1"/1 -> Sum/2
  Saturation/1 -> Bus Creator1/1, Mux/3  "current [A]"
  Saturation1/1 -> Product/3

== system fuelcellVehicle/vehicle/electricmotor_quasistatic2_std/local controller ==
  cmd in : Inport  OutDataType=sfix(16)  OutScaling=2^0
  sensor in : Inport  Port=2  OutDataType=sfix(16)  OutScaling=2^0
  Bus Creator1 : BusCreator  Inputs=1
  Bus Creator2 : BusCreator  Inputs=3
  Bus Selector1 : BusSelector  OutputSignals=speedref [rad/s],select [0;1],torqueref [Nm]
  Bus Selector3 : BusSelector  OutputSignals=voltage [V],speed [rad/s],em current [A]
  Gain : Gain  ParameterDataType=sfix(16)  ParameterScaling=2^0  OutDataType=sfix(16)  OutScaling=2^0
  Selector : Subsystem
  Speedcontroller : Subsystem
  Torquecontroller : Subsystem
  sensor out : Outport  OutDataType=sfix(16)  OutScaling=2^0
  ctrl out : Outport  Port=2  OutDataType=sfix(16)  OutScaling=2^0
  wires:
  cmd in/1 -> Bus Selector1/1
  Bus Selector1/1 -> Speedcontroller/1(Speedref)  "<speedref [rad/s]>"
  Bus Selector1/2 -> Selector/3(Select)  "<select [0;1]>"
  Bus Creator2/1 -> sensor out/1  "electricmotor"
  Selector/1(Ctrl) -> Bus Creator2/1, Bus Creator1/1  "voltage [V]"
  sensor in/1 -> Bus Selector3/1
  Bus Selector3/1 -> Selector/4(BatVolt)  "<voltage [V]>"
  Bus Selector3/3 -> Gain/1  "<em current [A]>"
  Bus Creator1/1 -> ctrl out/1
  Bus Selector1/3 -> Torquecontroller/1(Torqueref)  "<torqueref [Nm]>"
  Bus Selector3/2 -> Speedcontroller/2(Speed), Bus Creator2/2, Torquecontroller/2(Speed), Selector/5(Speed [rad/s])  "<speed [rad/s]>"
  Torquecontroller/1(Volt) -> Selector/2(TorqueCtrl)
  Speedcontroller/1(Volt) -> Selector/1(SpeedCtrl)
  Gain/1 -> Bus Creator2/3  "current [A]"

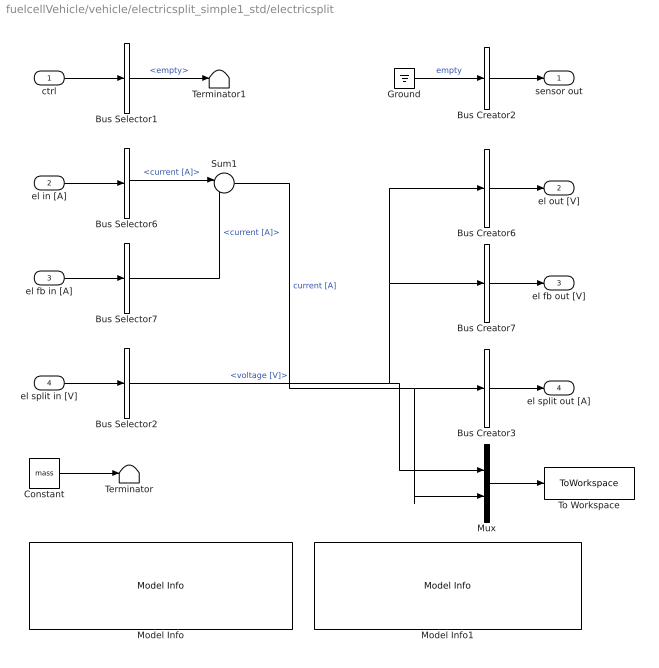
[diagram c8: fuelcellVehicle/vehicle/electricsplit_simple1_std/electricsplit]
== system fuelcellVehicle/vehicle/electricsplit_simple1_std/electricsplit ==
  ctrl : Inport  OutDataType=sfix(16)  OutScaling=2^0
  el in [A] : Inport  Port=2  OutDataType=sfix(16)  OutScaling=2^0
  el fb in [A] : Inport  Port=3  OutDataType=sfix(16)  OutScaling=2^0
  el split in [V] : Inport  Port=4  OutDataType=sfix(16)  OutScaling=2^0
  Bus Creator{2..3,6..7} (4 alike) : BusCreator  Inputs=1
  Bus Selector1 : BusSelector  OutputSignals=empty
  Bus Selector2 : BusSelector  OutputSignals=voltage [V]
  Bus Selector6 : BusSelector  OutputSignals=current [A]
  Bus Selector7 : BusSelector  OutputSignals=current [A]
  Constant : Constant  Value=mass  OutDataType=sfix(16)  OutScaling=2^0
  Ground : Ground
  Model Info : simulink/Model-Wide Utilities/Model Info  SystemSampleTime=-1  InitialBlockCM=None  BlockCM=None  Frame=on  DisplayStringWithTags=|  HorizontalTextAlignment=Left  LeftAlignmentValue=0.02  SourceBlockDiagram=fuelcellVehicle  TagMaxNumber=20
      | Modified: %<ModifiedDate>
      | 
      | The nodes "ctrl" and "sensor out" must conform 
      | with the corresponding nodes of the local controller. 
      | The other nodes are fixed.
  Model Info1 : simulink/Model-Wide Utilities/Model Info  SystemSampleTime=-1  InitialBlockCM=None  BlockCM=None  Frame=on  DisplayStringWithTags=Your own comments!  HorizontalTextAlignment=Left  LeftAlignmentValue=0.02  SourceBlockDiagram=fuelcellVehicle  TagMaxNumber=20
  Mux : Mux  Inputs=2
  Sum1 : Sum  Inputs=|-+  OutDataType=sfix(16)  OutScaling=2^0
  Terminator : Terminator
  Terminator1 : Terminator
  To Workspace : ToWorkspace  VariableName=electricsplit_simple1_std  SampleTime=-1  SaveFormat=Array
  sensor out : Outport  OutDataType=sfix(16)  OutScaling=2^0
  el out [V] : Outport  Port=2  OutDataType=sfix(16)  OutScaling=2^0
  el fb out [V] : Outport  Port=3  OutDataType=sfix(16)  OutScaling=2^0
  el split out [A] : Outport  Port=4  OutDataType=sfix(16)  OutScaling=2^0
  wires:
  Constant/1 -> Terminator/1
  Bus Selector2/1 -> Bus Creator6/1, Bus Creator7/1, Mux/1  "<voltage [V]>"
  Bus Creator3/1 -> el split out [A]/1
  Bus Creator2/1 -> sensor out/1
  ctrl/1 -> Bus Selector1/1
  Bus Selector1/1 -> Terminator1/1  "<empty>"
  el in [A]/1 -> Bus Selector6/1
  Bus Selector6/1 -> Sum1/1  "<current [A]>"
  Bus Creator6/1 -> el out [V]/1
  el fb in [A]/1 -> Bus Selector7/1
  Bus Selector7/1 -> Sum1/2  "<current [A]>"
  Bus Creator7/1 -> el fb out [V]/1
  Sum1/1 -> Bus Creator3/1, Mux/2  "current [A]"
  el split in [V]/1 -> Bus Selector2/1
  Ground/1 -> Bus Creator2/1  "empty"
  Mux/1 -> To Workspace/1

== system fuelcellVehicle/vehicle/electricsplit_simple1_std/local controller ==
  sensor in : Inport  OutDataType=sfix(16)  OutScaling=2^0
  Bus Creator1 : BusCreator  Inputs=1
  Bus Selector2 : BusSelector  OutputSignals=empty
  Ground : Ground
  Model Info : simulink/Model-Wide Utilities/Model Info  SystemSampleTime=-1  InitialBlockCM=None  BlockCM=None  Frame=on  DisplayStringWithTags=|  HorizontalTextAlignment=Left  LeftAlignmentValue=0.02  SourceBlockDiagram=fuelcellVehicle  TagMaxNumber=20
      | Modified: %<ModifiedDate>
      | The node "sensor out" is fixed.
      | The nodes "sensor in" and "ctrl", however, 
      | may be adjusted arbitrarily since the local controller is 
      | made specifically for a certain component model.
  Model Info1 : simulink/Model-Wide Utilities/Model Info  SystemSampleTime=-1  InitialBlockCM=None  BlockCM=None  Frame=on  DisplayStringWithTags=Your own comments!  HorizontalTextAlignment=Left  LeftAlignmentValue=0.02  SourceBlockDiagram=fuelcellVehicle  TagMaxNumber=20
  Terminator1 : Terminator
  ctrl : Outport  OutDataType=sfix(16)  OutScaling=2^0
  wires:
  Bus Creator1/1 -> ctrl/1
  Ground/1 -> Bus Creator1/1  "empty"
  sensor in/1 -> Bus Selector2/1
  Bus Selector2/1 -> Terminator1/1  "<empty>"

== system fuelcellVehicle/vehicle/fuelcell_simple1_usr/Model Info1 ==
  EmptySubsystem : Subsystem

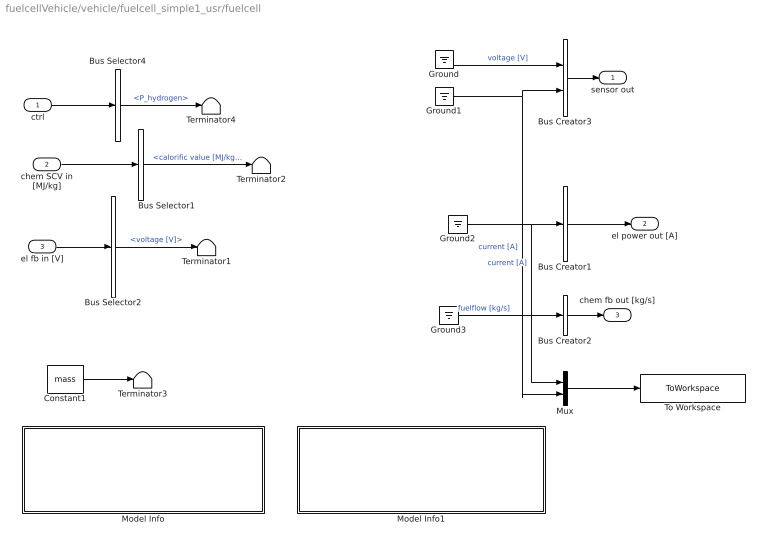
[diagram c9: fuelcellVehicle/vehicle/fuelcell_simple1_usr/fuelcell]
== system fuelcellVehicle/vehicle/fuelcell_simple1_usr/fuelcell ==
  ctrl : Inport  OutDataType=sfix(16)  OutScaling=2^0
  chem SCV in [MJ/kg] : Inport  Port=2  OutDataType=sfix(16)  OutScaling=2^0
  el fb in [V] : Inport  Port=3  OutDataType=sfix(16)  OutScaling=2^0
  Bus Creator1 : BusCreator  Inputs=1
  Bus Creator2 : BusCreator  Inputs=1
  Bus Creator3 : BusCreator  Inputs=2
  Bus Selector1 : BusSelector  OutputSignals=calorific value [MJ/kg]
  Bus Selector2 : BusSelector  OutputSignals=voltage [V]
  Bus Selector4 : BusSelector  OutputSignals=P_hydrogen
  Constant1 : Constant  Value=mass  OutDataType=sfix(16)  OutScaling=2^0
  Ground{,1..3} (4 alike) : Ground
  Model Info : Subsystem  LoadFcn=slcm LoadBlock;  InitFcn=slcm('UpdateAllCMBlocksInThisModelInit')  mask(CMBlock){InitialSaveTempField=, InitialBlockCM=None, BlockCM=None, Frame=on, SaveTempField=, DisplayStringWithTags=Modified: %<ModifiedDate>  The nodes "ctrl" and "sensor out" must conform  with the corresponding nodes of the local controller.  The other nodes are fixed., MaskDisplayString=Modified: Fri Dec  3 15:47:20 2010\n\nThe nodes "ctrl" and "sensor out" must conform \nwith the corresponding nodes of the local controller. \nThe other nodes are fixed., HorizontalTextAlignment=Left, LeftAlignmentValue=0.02, SourceBlockDiagram=fuelcellVehicle, TagMaxNumber=20, CMTag1=, CMTag2=, CMTag3=, CMTag4=, CMTag5=, CMTag6=, CMTag7=, CMTag8=, CMTag9=, CMTag10=, CMTag11=, CMTag12=, CMTag13=, CMTag14=, CMTag15=, CMTag16=, CMTag17=, CMTag18=, CMTag19=, CMTag20=}
      mask help: This block allows revision control information to be displayed within the model.
  Model Info1 : Subsystem  LoadFcn=slcm LoadBlock;  InitFcn=slcm('UpdateAllCMBlocksInThisModelInit')  mask(CMBlock){InitialSaveTempField=, InitialBlockCM=None, BlockCM=None, Frame=on, SaveTempField=, DisplayStringWithTags=Your own comments!, MaskDisplayString=Your own comments!, HorizontalTextAlignment=Left, LeftAlignmentValue=0.02, SourceBlockDiagram=fuelcellVehicle, TagMaxNumber=20, CMTag1=, CMTag2=, CMTag3=, CMTag4=, CMTag5=, CMTag6=, CMTag7=, CMTag8=, CMTag9=, CMTag10=, CMTag11=, CMTag12=, CMTag13=, CMTag14=, CMTag15=, CMTag16=, CMTag17=, CMTag18=, CMTag19=, CMTag20=}
      mask help: This block allows revision control information to be displayed within the model.
  Mux : Mux  Inputs=2
  Terminator{1..4} (4 alike) : Terminator
  To Workspace : ToWorkspace  VariableName=fuelcell_simple1_usr  SampleTime=-1  SaveFormat=Array
  sensor out : Outport  OutDataType=sfix(16)  OutScaling=2^0
  el power out [A] : Outport  Port=2  OutDataType=sfix(16)  OutScaling=2^0
  chem fb out [kg/s] : Outport  Port=3  OutDataType=sfix(16)  OutScaling=2^0
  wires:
  el fb in [V]/1 -> Bus Selector2/1
  Bus Creator1/1 -> el power out [A]/1
  Bus Creator3/1 -> sensor out/1
  ctrl/1 -> Bus Selector4/1
  chem SCV in [MJ/kg]/1 -> Bus Selector1/1
  Ground3/1 -> Bus Creator2/1  "fuelflow [kg/s]"
  Constant1/1 -> Terminator3/1
  Bus Creator2/1 -> chem fb out [kg/s]/1
  Mux/1 -> To Workspace/1
  Bus Selector4/1 -> Terminator4/1  "<P_hydrogen>"
  Bus Selector2/1 -> Terminator1/1  "<voltage [V]>"
  Bus Selector1/1 -> Terminator2/1  "<calorific value [MJ/kg]>"
  Ground/1 -> Bus Creator3/1  "voltage [V]"
  Ground1/1 -> Bus Creator3/2, Mux/2  "current [A]"
  Ground2/1 -> Bus Creator1/1, Mux/1  "current [A]"

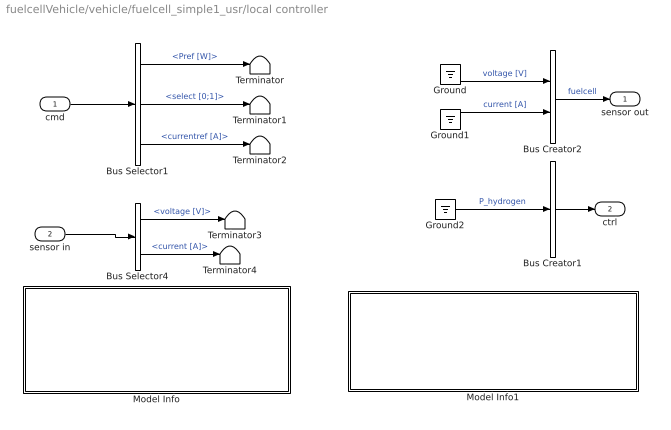
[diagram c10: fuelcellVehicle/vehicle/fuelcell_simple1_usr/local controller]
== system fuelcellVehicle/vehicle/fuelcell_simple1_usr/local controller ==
  cmd : Inport  OutDataType=sfix(16)  OutScaling=2^0
  sensor in : Inport  Port=2  OutDataType=sfix(16)  OutScaling=2^0
  Bus Creator1 : BusCreator  Inputs=1
  Bus Creator2 : BusCreator  Inputs=2
  Bus Selector1 : BusSelector  OutputSignals=Pref [W],select [0;1],currentref [A]
  Bus Selector4 : BusSelector  OutputSignals=voltage [V],current [A]
  Ground : Ground
  Ground1 : Ground
  Ground2 : Ground
  Model Info : Subsystem  LoadFcn=slcm LoadBlock;  InitFcn=slcm('UpdateAllCMBlocksInThisModelInit')  mask(CMBlock){InitialSaveTempField=, InitialBlockCM=None, BlockCM=None, Frame=on, SaveTempField=, DisplayStringWithTags=Modified: %<ModifiedDate> The nodes "cmd" and "sensor out" are fixed. The "select" signal defines whether the upper  (=1) or lower (=0) signal is used. The nodes "sensor in" and "ctrl", however,  may be adjusted arbitrarily since the local  controller is made specifically for a certain  component model., MaskDisplayString=Modified: Fri Dec  3 15:47:20 2010\nThe nodes "cmd" and "sensor out" are fixed.\nThe "select" signal defines whether the upper \n(=1) or lower (=0) signal is used.\nThe nodes "sensor in" and "ctrl", however, \nmay be adjusted arbitrarily since the local \ncontroller is made specifically for a certain \ncomponent model., HorizontalTextAlignment=Left, LeftAlignmentValue=0.02, SourceBlockDiagram=fuelcellVehicle, TagMaxNumber=20, CMTag1=, CMTag2=, CMTag3=, CMTag4=, CMTag5=, CMTag6=, CMTag7=, CMTag8=, CMTag9=, CMTag10=, CMTag11=, CMTag12=, CMTag13=, CMTag14=, CMTag15=, CMTag16=, CMTag17=, CMTag18=, CMTag19=, CMTag20=}
      mask help: This block allows revision control information to be displayed within the model.
  Model Info1 : Subsystem  LoadFcn=slcm LoadBlock;  InitFcn=slcm('UpdateAllCMBlocksInThisModelInit')  mask(CMBlock){InitialSaveTempField=, InitialBlockCM=None, BlockCM=None, Frame=on, SaveTempField=, DisplayStringWithTags=Your own comments!, MaskDisplayString=Your own comments!, HorizontalTextAlignment=Left, LeftAlignmentValue=0.02, SourceBlockDiagram=fuelcellVehicle, TagMaxNumber=20, CMTag1=, CMTag2=, CMTag3=, CMTag4=, CMTag5=, CMTag6=, CMTag7=, CMTag8=, CMTag9=, CMTag10=, CMTag11=, CMTag12=, CMTag13=, CMTag14=, CMTag15=, CMTag16=, CMTag17=, CMTag18=, CMTag19=, CMTag20=}
      mask help: This block allows revision control information to be displayed within the model.
  Terminator{,1..4} (5 alike) : Terminator
  sensor out : Outport  OutDataType=sfix(16)  OutScaling=2^0
  ctrl : Outport  Port=2  OutDataType=sfix(16)  OutScaling=2^0
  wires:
  Bus Creator1/1 -> ctrl/1
  Bus Creator2/1 -> sensor out/1  "fuelcell"
  sensor in/1 -> Bus Selector4/1
  Bus Selector1/2 -> Terminator1/1  "<select [0;1]>"
  Bus Selector1/1 -> Terminator/1  "<Pref [W]>"
  Bus Selector1/3 -> Terminator2/1  "<currentref [A]>"
  cmd/1 -> Bus Selector1/1
  Ground2/1 -> Bus Creator1/1  "P_hydrogen"
  Ground1/1 -> Bus Creator2/2  "current [A]"
  Ground/1 -> Bus Creator2/1  "voltage [V]"
  Bus Selector4/1 -> Terminator3/1  "<voltage [V]>"
  Bus Selector4/2 -> Terminator4/1  "<current [A]>"

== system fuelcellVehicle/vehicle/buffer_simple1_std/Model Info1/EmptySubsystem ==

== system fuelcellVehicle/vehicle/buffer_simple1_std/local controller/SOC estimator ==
  current in : Inport  OutDataType=sfix(16)  OutScaling=2^0
  Gain : Gain  Gain=1/Emax_c  ParameterDataType=sfix(16)  ParameterScaling=2^0  OutDataType=sfix(16)  OutScaling=2^0
  Inner Resistance : Gain  Gain=Ri_c  ParameterDataType=sfix(16)  ParameterScaling=2^0  OutDataType=sfix(16)  OutScaling=2^0
  Inner Resistance1 : Gain  Orientation=left  Gain=Kvol_c  ParameterDataType=sfix(16)  ParameterScaling=2^0  OutDataType=sfix(16)  OutScaling=2^0
  Integrator : Integrator  InitialCondition=SOCinit_c  LimitOutput=on  UpperSaturationLimit=1  LowerSaturationLimit=0
  Math Function : Math  Operator=square  OutDataType=sfix(16)  OutScaling=2^0
  Product : Product  OutDataType=sfix(16)  OutScaling=2^0
  Sum : Sum  Inputs=-|-  OutDataType=sfix(16)  OutScaling=2^0
  SOC : Outport  OutDataType=sfix(16)  OutScaling=2^0
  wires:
  Integrator/1 -> SOC/1, Inner Resistance1/1
  Gain/1 -> Integrator/1
  current in/1 -> Math Function/1, Product/1
  Math Function/1 -> Inner Resistance/1
  Inner Resistance1/1 -> Product/2
  Inner Resistance/1 -> Sum/1
  Product/1 -> Sum/2
  Sum/1 -> Gain/1
